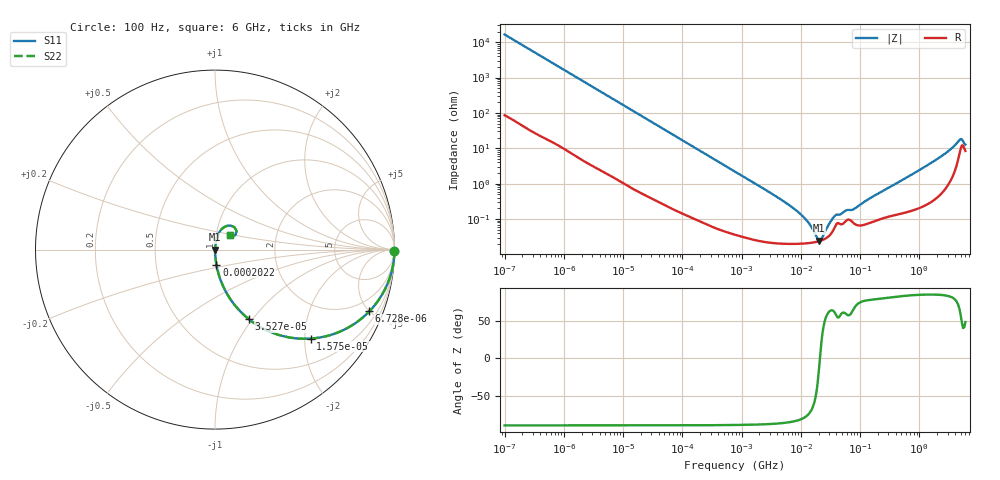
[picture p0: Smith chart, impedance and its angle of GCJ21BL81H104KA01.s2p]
!Murata Part Number: GCJ21BL81H104KA01
!These Parameters are Measured in Series Mode Connection
!Data Generated on Mar 13, 2026
!  o--ll--o
!Port1  Port2
!  o------o
!Operation Temp=25[degC], DC Bias Voltage=0[V]
!Freq. Start=100[Hz] Stop=6[GHz] 401[Steps]
# Hz S RI R 50
!Freq.(Hz) S11(Real) S11(Imag) S21(Real) S21(Imag) S12(Real) S12(Imag) S22(Real) S22(Imag)
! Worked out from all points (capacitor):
!   401 points, 100 Hz to 6 GHz, reference 50 ohm
!   read as one part in series: C = 96.3 nF near 109 Hz
!   lowest |Z| = 24.3 mohm at 20.35 MHz (marker M1)
!   series resonance near 21.01 MHz, so ESL is about 600 pH
!   S11 on the Smith chart (normalised r, x): 100 Hz: open; 6.728 kHz: 1.03, -4.98; 15.75 kHz: 1.01, -2.13; 35.27 kHz: 1.01, -0.96; 202.2 kHz: 1.00, -0.17; 6 GHz: 1.17, +0.19
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100  0.9999 -0.00606  6.83e-05 0.00606  6.83e-05 0.00606  0.9999 -0.00606
627  0.9984 -0.0377  0.00164 0.0377  0.00164 0.0377  0.9984 -0.0377
2008  0.9851 -0.1185  0.0149 0.1185  0.0149 0.1185  0.9851 -0.1185
6728  0.8597 -0.3442  0.1403 0.3442  0.1403 0.3442  0.8597 -0.3442
15752  0.5324 -0.4958  0.4676 0.4958  0.4676 0.4958  0.5324 -0.4958
35265  0.1879 -0.3871  0.8121 0.3871  0.8121 0.3871  0.1879 -0.3871
40335  0.1508 -0.3543  0.8492 0.3543  0.8492 0.3543  0.1508 -0.3543
75495  0.0494 -0.2127  0.9506 0.2127  0.9506 0.2127  0.0494 -0.2127
202169  0.00785 -0.0834  0.9921 0.0834  0.9921 0.0834  0.00785 -0.0834
774597  0.000847 -0.0221  0.9992 0.0221  0.9992 0.0221  0.000847 -0.0221
6948629  0.000203 -0.00222  0.9998 0.00222  0.9998 0.00222  0.000203 -0.00222
1.137099e7  0.000205 -0.00108  0.9998 0.00108  0.9998 0.00108  0.000205 -0.00108
1.555665e7  0.000216 -0.000508  0.9998 0.000508  0.9998 0.000508  0.000216 -0.000508
2.035112e7  0.000237 -5.32e-05  0.9998 5.32e-05  0.9998 5.32e-05  0.000237 -5.32e-05
2.225763e7  0.000249 9.89e-05  0.9998 -9.89e-05  0.9998 -9.89e-05  0.000249 9.89e-05
3.045065e7  0.000342 0.000673  0.9997 -0.000673  0.9997 -0.000673  0.000342 0.000673
3.80911e7  0.000625 0.0011  0.9994 -0.0011  0.9994 -0.0011  0.000625 0.0011
7.797396e7  0.000768 0.00174  0.9992 -0.00174  0.9992 -0.00174  0.000768 0.00174
3.124326e8  0.00124 0.00778  0.9988 -0.00778  0.9988 -0.00778  0.00124 0.00778
2.048624e9  0.0067 0.0503  0.9933 -0.0503  0.9933 -0.0503  0.0067 0.0503
4.796499e9  0.0873 0.1338  0.9127 -0.1338  0.9127 -0.1338  0.0873 0.1338
6e9  0.0847 0.0807  0.9153 -0.0807  0.9153 -0.0807  0.0847 0.0807
